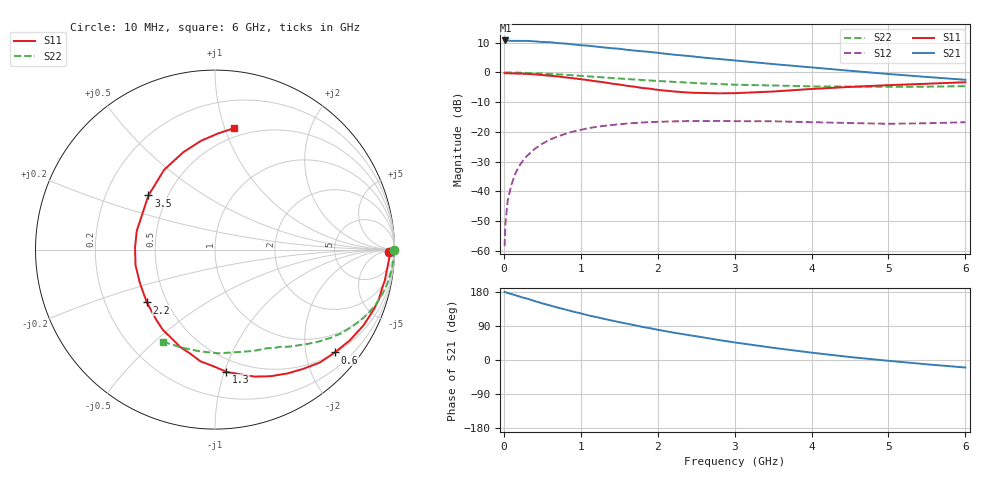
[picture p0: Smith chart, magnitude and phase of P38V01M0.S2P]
! SIEMENS Small Signal Semiconductors
! BFP181
! Si NPN RF Bipolar Junction Transistor in SOT143
! VCE = 8 V  IC = 1 mA
! Common Emitter S-Parameters:  March  1996
# GHz  S  MA  R  50
!  f  S11  S21  S12  S22
! GHz  MAG  ANG  MAG  ANG  MAG  ANG  MAG  ANG
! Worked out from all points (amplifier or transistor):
!   36 points, 10 MHz to 6 GHz, reference 50 ohm
!   highest |S21| = 10.8 dB at 20 MHz (marker M1)
!   |S21| within 3 dB of that: start of sweep to 1.558 GHz
!   unconditionally stable (mu >= 1): 3.249 GHz to end of sweep
!   at 250 MHz: K = 0.09, MSG = 20.1 dB, |S12| = -29.6 dB
!   at 1.4 GHz: K = 0.48, MSG = 12.9 dB, |S12| = -17.7 dB
!   at 6 GHz: K = 1.26, MAG = 4.1 dB, |S12| = -16.7 dB
!   lowest NFmin = 1.30 dB at 450 MHz
!   S11 on the Smith chart (normalised r, x): 10 MHz: 57, -23; 600 MHz: 0.51, -2.61; 1.3 GHz: 0.40, -1.02; 2.2 GHz: 0.39, -0.30; 3.5 GHz: 0.39, +0.31; 6 GHz: 0.42, +1.08
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0.01  0.9706 -0.7  3.448 179.5  0.0012 87.0  0.9978 -0.2
0.02  0.9742 -1.3  3.452 179.3  0.0028 83.5  0.9972 -0.7
0.05  0.9711 -3.2  3.43 176.9  0.007 91.4  0.9968 -1.6
0.1  0.9641 -7.0  3.399 174.0  0.0131 84.3  0.9956 -3.3
0.2  0.9549 -13.8  3.404 167.7  0.0268 80.5  0.9909 -6.5
0.3  0.9455 -20.6  3.397 162.2  0.0394 76.2  0.9834 -9.7
0.4  0.9287 -27.1  3.334 155.5  0.0518 71.7  0.9732 -12.8
0.6  0.8801 -40.6  3.227 143.9  0.0743 63.2  0.9463 -18.9
0.8  0.8261 -53.6  3.061 133.1  0.0928 55.0  0.913 -24.3
1.1  0.7415 -72.6  2.819 117.7  0.1158 44.8  0.8595 -31.4
1.3  0.6839 -84.7  2.636 108.8  0.1263 38.4  0.8239 -35.7
1.5  0.6273 -97.5  2.504 99.9  0.1343 33.1  0.7896 -39.4
1.8  0.5482 -116.7  2.268 87.4  0.1442 26.3  0.7467 -44.3
2.2  0.4806 -142.2  1.996 72.5  0.1504 18.5  0.696 -50.5
2.4  0.4582 -155.9  1.893 65.8  0.1522 15.1  0.6747 -53.4
2.8  0.4456 178.3  1.682 52.6  0.1528 9.7  0.6395 -59.0
3  0.4482 166.6  1.593 46.4  0.1517 7.3  0.6225 -61.9
3.5  0.4781 140.9  1.384 32.2  0.151 2.7  0.6034 -69.4
4  0.5276 122.4  1.216 19.4  0.1458 -0.3  0.5838 -78.2
4.5  0.5712 107.9  1.067 7.8  0.1412 -2.5  0.578 -88.1
5.5  0.6463 88.7  0.84 -11.4  0.14 0.0  0.5768 -108.6
6  0.6848 81.1  0.753 -19.8  0.1454 0.6  0.5887 -119.3
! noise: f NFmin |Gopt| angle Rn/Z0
0.45  1.3  0.7  18  0.5
0.9  1.4  0.6  39  0.52
1.8  1.85  0.4  81  0.47
